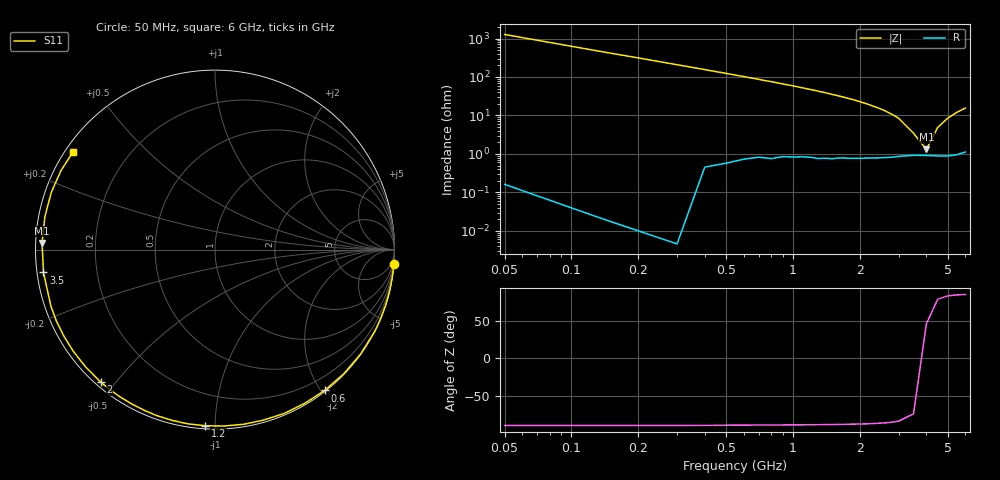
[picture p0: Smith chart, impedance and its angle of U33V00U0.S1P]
! SIEMENS Discrete & RF Semiconductors
! BBY53-02W
! Si Tuning Diode in SCD-80
! VR = 3 V
! S-Parameters:  September  1997
# GHz  S  MA  R  50
!  f  S11
! GHz  MAG  ANG
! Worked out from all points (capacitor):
!   34 points, 50 MHz to 6 GHz, reference 50 ohm
!   read as one part to ground: C = 2.53 pF near 50 MHz
!   lowest |Z| = 1.32 ohm at 4 GHz (marker M1)
!   series resonance near 3.888 GHz, so ESL is about 660 pH
!   S11 on the Smith chart (normalised r, x): 50 MHz: 0, -25; 600 MHz: 0.01, -2.05; 1.2 GHz: 0.02, -0.95; 2 GHz: 0.02, -0.46; 3.5 GHz: 0.02, -0.07; 6 GHz: 0.02, +0.31
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0.05  1 -4.5
0.1  1 -9.1
0.2  1 -18.1
0.3  1 -27.0
0.4  0.9983 -35.6
0.5  0.9968 -44.0
0.6  0.9944 -52.1
0.7  0.9919 -59.8
0.8  0.9908 -67.2
0.9  0.9876 -74.3
1  0.9861 -80.8
1.1  0.9841 -87.2
1.2  0.9828 -93.2
1.4  0.9809 -104.2
1.6  0.9782 -114.0
1.8  0.9766 -122.8
2  0.975 -130.7
2.2  0.973 -138.0
2.4  0.9718 -144.4
2.6  0.9704 -150.4
2.8  0.9691 -155.9
3  0.9669 -161.0
3.5  0.964 -172.4
4  0.9642 177.8
4.5  0.9654 169.0
5  0.9663 160.7
5.5  0.9645 152.8
6  0.9598 145.5
